(* Logix 5000 DataType export JVL_AXIS_MAC; software revision 33.00 *)

TYPE JVL_AXIS_MAC :   // Drive Data
STRUCT
   ActualMode : DINT;   // actual Mode
   ActualPosition : REAL;   // P_IST
   ActualVelocity : REAL;   // V_IST(16)
   ActualTorque : REAL;   // ACTUAL_TORQUE
   AxisStatusError : JVL_MAC_Status_Error;   // Holds an indication of which error that is detected
   Home_Mode : DINT;   // Homemode
   RequestedMode : DINT;   // requested Mode
   RequestedPosition : REAL;   // P_SOLL
   RequestedVelocity : REAL;   // V_SOLL
   RequestedAcceleration : REAL;   // A_SOLL
   GeneralCommand : DINT;
   CommandTorque : REAL;   // Requested Torque, T_SOLL
   ZeroSearchVelocity : REAL;   // Homing velocity
   ZeroSearchPosition : REAL;   // Homing position
   ZeroSearchTorque : DINT;   // Homing torque setpoint threshold value
   ZeroSearchTThreshold : DINT;   // Threshold for torque zerosearch trigger, usually 20% lower than running torque
   TravelConst : REAL;   // Factor to multiply P_IST and P_SOLL for scaling
   VelConst : REAL;   // Factor to multiply V_SOLL and V_IST to get scaled velocity value
   HomingType : DINT;   // Holds the reqested homingtype
   LoadFactor : DINT;   // Inertia ratio motor/load
   MotorType : DINT;   // MotorType configured. 0=No Selection 1=MAC50-141-A/K (old) 2=MAC50-141-F (new), MAC400, 402, 1500, 3000, 4500 (All Encoder variations) 3=MAC800 with incremental encoder 4=MAC800 with abs. encoder
   Configured : DINT;
   MSG_OutValue : DINT;   // Used in exp. output message to the motor
   MSG_InValue : DINT;   // Used in Exp. output message, to get value from motor
   MSG_OutInstance : DINT;   // Registernumber
   MSG_InInstance : DINT;   // Registernummer
   V_SOLL_CountsPerSample : REAL;
   A_SOLL_CountsPerSample2 : REAL;
   AOI_Type : DINT;   // MAC_Disable = 1, MAC_Home = 2, MAC_Jog = 3, MAC_Position = 4, MAC_Reset = 5, MAC_Stop = 6
   Position_AppType : REAL;   // calculated Position by Application Type
   MSG_Out_Execute : BOOL;   // Enable MSG_Out
   MSG_In_Execute : BOOL;   // Enable MSG_In
   ErrorReset : BOOL;
   MSG_Out_Busy : BOOL;
   MSG_In_Busy : BOOL;
   MSG_Out_Done : BOOL;
   MSG_In_Done : BOOL;
END_STRUCT
END_TYPE

TYPE JVL_MAC_Status_Error :   // Axis Faults Status
STRUCT
   Error : BOOL;
   InitialisationError : BOOL;
   FlashMemoryError : BOOL;
   STOError : BOOL;
   NotUsed_2 : BOOL;
   NotUsed_3 : BOOL;
   OUT1 : BOOL;
   OUT2 : BOOL;
   NotUsed : BOOL;
   ControlVoltageError : BOOL;
   ShortCircuitError : BOOL;
   MotorSupplyDetected : BOOL;
   MotorLocked : BOOL;
   CommsError : BOOL;
   CurrentLoopError : BOOL;
   ModbusSlaveError : BOOL;
   TemperatureError : BOOL;
   UndervoltageError : BOOL;
   UndervoltageDetect : BOOL;
   OvervoltageError : BOOL;
   OvercurrentError : BOOL;
   OverspeedError : BOOL;
   AllowExceedingOfSoftwareLimits : BOOL;
   EncoderError : BOOL;
   I2TError : BOOL;
   FollowingError : BOOL;
   FunctionError : BOOL;
   BreakingResistorOverTempError : BOOL;
   InPosition : BOOL;
   Accelerating : BOOL;
   Decelerating : BOOL;
   SoftwareLimitExceeded : BOOL;
END_STRUCT
END_TYPE
